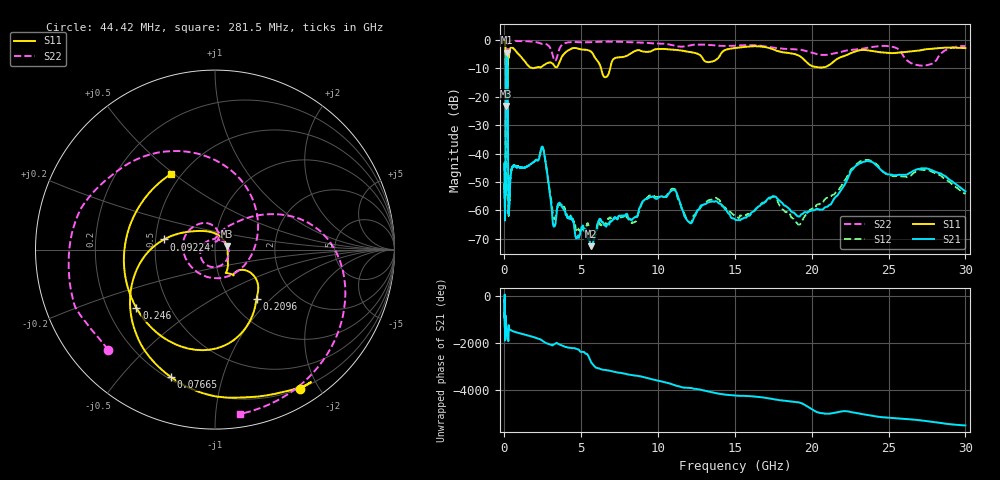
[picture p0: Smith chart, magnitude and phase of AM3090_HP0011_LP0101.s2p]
! Date/Time: Thu, Feb 28, 2019 1:56 PM
! Network Analyzer: Agilent Technologies E8364B Rev: A.07.50.67
! Sweep from 0.010 to 30.000 GHz, 1601 Points, Sweep Type: LOG
! Power Supply: 5.023 V, 0.002 A
# Hz S DB R 50
!freq MagS11 AngS11 MagS21 AngS21 MagS12 AngS12 MagS22 AngS22
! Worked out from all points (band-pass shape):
!   1601 points, 10 MHz to 30 GHz, reference 50 ohm
!   highest |S21| = -4.40 dB at 144 MHz (marker M1); lowest = -72.6 dB at 5.64 GHz (marker M2)
!   |S21| within 3 dB of the highest: 102.2 MHz to 201.5 MHz (99.36 MHz wide, 65.4 % of centre)
!   lowest |S11| = -23.2 dB at 100.4 MHz (marker M3), VSWR 1.15, Z = 57.1 + j2.07 ohm
!   |S11| at or under -10 dB: 91.74 MHz to 202.8 MHz (111.1 MHz wide, 75.4 % of centre); 6.288 GHz to 6.877 GHz (588.9 MHz wide, 8.95 % of centre)
!   |S22| runs from -27.2 to -0.1 dB; largest |S21 - S12| = 0.012
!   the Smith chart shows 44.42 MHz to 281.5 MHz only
!   S11 on the Smith chart (normalised r, x): 44.42 MHz: 0.19, -1.76; 76.65 MHz: 0.21, -0.69; 92.24 MHz: 0.55, +0.07; 209.6 MHz: 1.31, -0.82; 246 MHz: 0.32, -0.30; 281.5 MHz: 0.44, +0.49
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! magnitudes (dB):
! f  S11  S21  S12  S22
! 10 MHz  -0.2  -46.0  -43.1  -0.6
! 38.04 MHz  -0.5  -62.4  -62.3  -1.4
! 44.42 MHz  -0.8  -56.8  -56.1  -1.8
! 76.65 MHz  -2.5  -46.6  -49.1  -4.6
! 92.24 MHz  -10.8  -15.4  -15.3  -15.9
! 100.4 MHz  -23.2  -8.0  -8.0  -14.8
! 144 MHz  -15.6  -4.4  -4.4  -23.0
! 144.7 MHz  -15.6  -4.4  -4.4  -22.8
! 209.6 MHz  -8.9  -9.7  -9.7  -14.3
! 246 MHz  -5.3  -53.7  -54.4  -1.5
! 281.5 MHz  -6.2  -61.0  -60.8  -0.7
! 550.5 MHz  -2.9  -44.5  -44.4  -0.2
! 2.084 GHz  -9.7  -42.4  -42.1  -0.8
! 2.533 GHz  -8.9  -38.5  -38.4  -1.3
! 3.22 GHz  -8.9  -65.6  -63.0  -6.9
! 3.613 GHz  -7.4  -57.6  -58.1  -2.7
! 5.64 GHz  -4.1  -72.6  -68.8  -0.8
! 7.926 GHz  -5.6  -61.4  -62.3  -0.7
! 10.76 GHz  -3.3  -53.6  -53.4  -1.6
! 19.41 GHz  -6.5  -61.3  -63.3  -3.6
! 23.48 GHz  -3.5  -42.8  -42.3  -2.9
! 30 GHz  -2.8  -53.3  -54.2  -2.1
